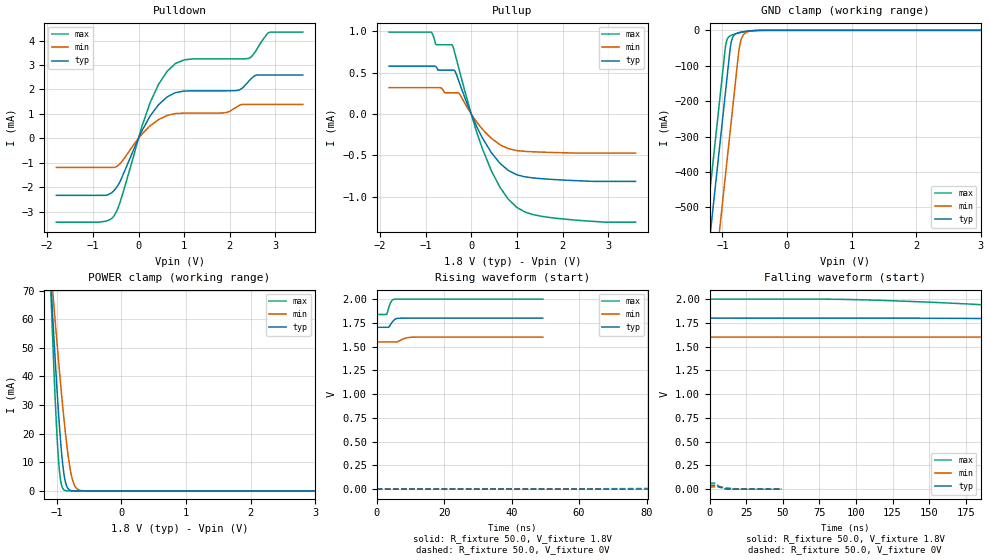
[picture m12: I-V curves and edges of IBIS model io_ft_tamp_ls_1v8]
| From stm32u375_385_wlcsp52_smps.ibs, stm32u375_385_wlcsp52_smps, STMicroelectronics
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[Model]   io_ft_tamp_ls_1v8
Model_type I/O
Polarity   Non-Inverting
Enable   Active-Low
| CAP_THRESHOLD on pad IOFT is "UDTCAPC" :
| Rising=30.0% of vddios   Falling=70.0% of vddios
| C_comp min and max val. don't necessarily correlate with the min and max pvt
| but are the smallest and greatest pad capacitance found.
| var   typ   min   max
C_comp   2.73010pF  2.72575pF  2.75285pF
|C_comp_pullup   1.48402pF  1.51992pF  1.63413pF
|C_comp_pulldown   1.24608pF  1.20583pF  1.11871pF
Vinl = 800.0mV
Vinh = 1.0V
Vmeas = 900.0mV   | Reference voltage for timing measurements
Cref  = 50.0pF   | Timing specification test load capacitance value
Rref  = 1.0MOhm   | Timing specification test load resistance value
Vref  = 990.0mV   | Timing specification test load voltage
[Model Spec]
| TIME_THRESHOLD on pin ZIV11 is "CMOS" :
| Rising=50.0% of vdd   Falling=50.0% of vdd
Vinl 694.50000mV 619.50000mV 778.50000mV
Vinh 1.08350V 957.50000mV 1.18750V
| variable   typ   min   max
[Temperature Range] 25.0 130.0 -40.0
| variable   typ   min   max
[Voltage Range] 1.8V 1.6V 2.0V
| variable   typ   min   max
[POWER Clamp Reference] 1.8V 1.6V 2.0V
| variable   typ   min   max
[GND Clamp Reference] 0V 0V 0V
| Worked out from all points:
|   slope of the pulldown table from 0 to 0.27 V, typ, clamps not added: 284 ohm
|   slope of the pullup table from 0 to 0.27 V, typ, clamps not added: 866 ohm
|   GND clamp passes 1 mA (typ) near -0.53 V on its own axis
|   POWER clamp passes 1 mA (typ) near -0.83 V on its own axis
|   rising waveform, R_fixture 50.0, V_fixture 1.8V: 20-80 % time 1.24ns typ, 2.05ns min, 927ps max; typ from 1.7 V to 1.8 V
|   falling waveform, R_fixture 50.0, V_fixture 1.8V: 20-80 % time 218ns typ, 387ns min, 140ns max; typ from 1.8 V to 1.7 V
[POWER Clamp]
-1.8V     399.1mA    292.1mA    557.7mA
-1.09V    71.2mA     76.8mA     67.14mA
-1.08V    67.05mA    73.98mA    61.2mA
-1.06V    58.89mA    68.38mA    49.67mA
-1.02V    43.22mA    57.4mA     28.67mA
-980mV    28.81mA    46.77mA    12.28mA
-940mV    16.45mA    36.61mA    3.257mA
-880mV    4.35mA     22.67mA    225.4uA
-820mV    610.4uA    11.29mA    13uA
-770mV    97.5uA     4.87mA     1.193uA
-640mV    753.5nA    196uA      2.462nA
3.6V      0A         0A         0A
[GND Clamp]
-1.8V     -1.614A    -1.849A    -1.484A
-1.3V     -764.3mA   -998.7mA   -634.2mA
-1.24V    -662.3mA   -896.7mA   -532.2mA
-1.05V    -339.3mA   -573.7mA   -209.2mA
-950mV    -169.3mA   -403.7mA   -42.69mA
-920mV    -118.3mA   -352.7mA   -23.09mA
-880mV    -51.11mA   -284.7mA   -15.46mA
-830mV    -16.2mA    -199.7mA   -11.8mA
-740mV    -6.183mA   -50.96mA   -7.241mA
-690mV    -4.389mA   -17.19mA   -5.148mA
-610mV    -2.335mA   -4.282mA   -2.511mA
3.6V      1.047nA    154.4nA    370.3pA
| variable   typ   min   max
[Pullup Reference] 1.8V 1.6V 2.0V
| variable   typ   min   max
[Pulldown Reference] 0V 0V 0V
[Pullup]
-1.8V     578.2uA    318.5uA    988.9uA
-880mV    578.2uA    318.5uA    988.1uA
-770mV    568.9uA    318.5uA    836.1uA
-420mV    529.3uA    256.8uA    835.1uA
-360mV    519.9uA    256.8uA    736.6uA
-270mV    393.1uA    249.8uA    545.6uA
30mV      -39.39uA   -25.35uA   -56.88uA
250mV     -293.7uA   -187.4uA   -427.6uA
630mV     -595.2uA   -370.9uA   -885.5uA
1V        -733.8uA   -441.7uA   -1.128mA
1.76V     -788.9uA   -463.8uA   -1.252mA
3.6V      -813.2uA   -472uA     -1.306mA
[Pulldown]
-1.8V     -2.333mA   -1.19mA    -3.431mA
-870mV    -2.333mA   -1.19mA    -3.431mA
-540mV    -2.142mA   -1.19mA    -3.179mA
-390mV    -1.711mA   -1.009mA   -2.535mA
250mV     900.6uA    504.7uA    1.44mA
440mV     1.376mA    767uA      2.21mA
810mV     1.868mA    1.014mA    3.062mA
2.12V     1.946mA    1.246mA    3.25mA
2.4V      2.301mA    1.387mA    3.263mA
2.58V     2.586mA    1.387mA    3.604mA
2.87V     2.591mA    1.387mA    4.337mA
3.6V      2.591mA    1.387mA    4.345mA
[Ramp]
dV/dt_r 23.66721mV/235.74885ns 13.81176mV/452.94978ns 37.8842mV/138.04935ns
dV/dt_f 58.29366mV/217.7165ns 31.01005mV/385.43584ns 97.50761mV/139.58407ns
R_load = 50.0
| Removed startup time: 0s 0s 0s  .
| Removed end time: 49.25ns.
[Rising Waveform]
R_fixture   = 50.0
V_fixture   = 1.8V
V_fixture_min = 1.6V
V_fixture_max = 2.0V
0s        1.703V     1.548V     1.837V
2.9ns     1.703V     1.548V     1.838V
3.55ns    1.705V     1.548V     1.909V
4.1ns     1.732V     1.548V     1.963V
4.65ns    1.761V     1.548V     1.99V
5.2ns     1.782V     1.548V     1.998V
6.8ns     1.799V     1.561V     2V
9.05ns    1.8V       1.593V     2V
11.05ns   1.8V       1.599V     2V
49.25ns   1.8V       1.6V       2V
| Removed startup time: 0s 0s 0s  .
| Removed end time: 2.49925us.
[Falling Waveform]
R_fixture   = 50.0
V_fixture   = 1.8V
V_fixture_min = 1.6V
V_fixture_max = 2.0V
0s        1.8V       1.6V       2V
102ns     1.8V       1.6V       1.994V
153ns     1.799V     1.6V       1.966V
200.4ns   1.793V     1.6V       1.928V
287.4ns   1.773V     1.599V     1.871V
362.9ns   1.748V     1.596V     1.85V
448.6ns   1.727V     1.591V     1.842V
629.9ns   1.709V     1.574V     1.838V
1.02us    1.703V     1.553V     1.837V
2.499us   1.703V     1.548V     1.837V
| Removed startup time: 0s 0s 0s  .
| Removed end time: 2.49925us.
[Rising Waveform]
R_fixture   = 50.0
V_fixture   = 0V
V_fixture_min = 0V
V_fixture_max = 0V
0s        14.15nV    218.7nV    13.56nV
51ns      -14.21uV   -6.659uV   452.4uV
102ns     441.9uV    -2.791uV   9.646mV
204ns     7.515mV    292.8uV    40.83mV
255.1ns   13.59mV    837.3uV    51.05mV
306.1ns   19.84mV    1.891mV    56.82mV
408.1ns   29.33mV    4.971mV    61.51mV
612.1ns   37.18mV    12.42mV    63.02mV
1.02us    39.34mV    20.63mV    63.13mV
2.499us   39.45mV    23.02mV    63.14mV
| Removed startup time: 0s 0s 0s  .
| Removed end time: 49.25ns.
[Falling Waveform]
R_fixture   = 50.0
V_fixture   = 0V
V_fixture_min = 0V
V_fixture_max = 0V
0s        39.45mV    23.04mV    63.15mV
3.7ns     39.44mV    23.04mV    62.95mV
4.4ns     38.96mV    23.04mV    54.69mV
6.05ns    29.39mV    23.03mV    34.19mV
7.7ns     20.49mV    22.48mV    17.21mV
9.7ns     11.31mV    18.12mV    6.962mV
11.6ns    5.969mV    14.25mV    1.05mV
15.1ns    770.3uV    8.017mV    204.6uV
24.15ns   58.91uV    569.8uV    13.33uV
49.25ns   2.081uV    9.402uV    4.501uV
